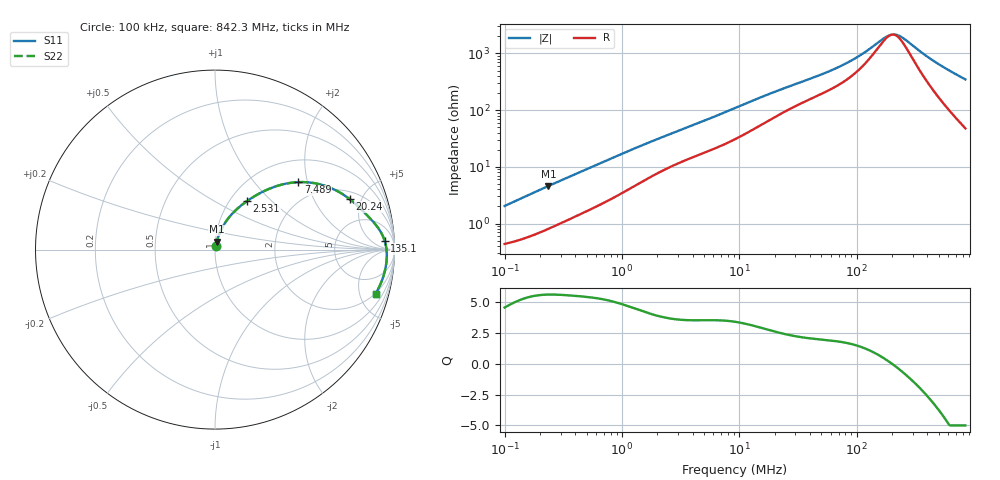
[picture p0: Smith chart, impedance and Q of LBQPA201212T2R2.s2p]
! LBQPA201212T2R2  S-PARAMETER MODEL  ( General Type )
! Model Generated by TAIYO YUDEN Corporation (http://www.ty-top.com)
! Version 1.0
! TAIYO YUDEN Control No. 191025NI43SB-FBB
! Copyright(c) 2019 TAIYO YUDEN CO.,LTD. All Rights Reserved.
! Product Description (link to TY-COMPAS)
! https://ds.yuden.co.jp/TYCOMPAS/or/detail?pn=LBQPA201212T2R2M&u=M
! Products Name : Inductors
! Characteristics :
!  Inductance : 2.2 uH , SRF(min) : 70 MHz , DC Resistance(max) : 0.429 Ohm
!  Rated Current : Saturation :530 mA , Temp Rise : 485 mA (20 degC)
!  Case Size : 2.0 x 1.25 / 0.079 x 0.049 [mm/inch] , Thickness : 1.25 / 0.049 [mm/inch]
!  (Conditions: Temperature = 25 degC , DC Bias Current/Voltage = 0A / 0V)
! External Node Assignments :
!  1  o---GGG---o  2
! GND o---------o GND
! Frequency Range : 0.1MHz  -  842.342835MHz  [ 402 STEP ]
# MHz S RI R 50
! Freq[MHz].  S11 Real  S11 Imag  S21 Real  S21 Imag  S12 Real  S12 Imag  S22 Real  S22 Imag
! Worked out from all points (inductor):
!   401 points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, 100 kHz to 842.3 MHz, reference 50 ohm
!   read as one part in series: L = 3.15 uH near 104.6 kHz
!   highest Q = 5.61 at 236 kHz (marker M1), where L = 3.05 uH
!   self-resonance near 199.7 MHz
!   S11 on the Smith chart (normalised r, x): 100 kHz: 1.01, +0.04; 2.531 MHz: 1.20, +0.72; 7.489 MHz: 1.50, +1.76; 20.24 MHz: 2.53, +3.97; 135.1 MHz: 19, +18; 842.3 MHz: 1.95, -6.91
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0.1  0.00474 0.0197  0.9953 -0.0197  0.9953 -0.0197  0.00474 0.0197
0.236005  0.00997 0.0444  0.99 -0.0444  0.99 -0.0444  0.00997 0.0444
0.454485  0.0212 0.0791  0.9788 -0.0791  0.9788 -0.0791  0.0212 0.0791
1.048642  0.0613 0.157  0.9387 -0.157  0.9387 -0.157  0.0613 0.157
2.065565  0.1428 0.2435  0.8572 -0.2435  0.8572 -0.2435  0.1428 0.2435
2.531409  0.1778 0.27  0.8222 -0.27  0.8222 -0.27  0.1778 0.27
4.354032  0.298 0.337  0.702 -0.337  0.702 -0.337  0.298 0.337
7.48895  0.4642 0.3759  0.5358 -0.3759  0.5358 -0.3759  0.4642 0.3759
9.177924  0.5333 0.3732  0.4667 -0.3732  0.4667 -0.3732  0.5333 0.3732
13.78451  0.6601 0.3369  0.3399 -0.3369  0.3399 -0.3369  0.6601 0.3369
20.24066  0.7498 0.2816  0.2502 -0.2816  0.2502 -0.2816  0.7498 0.2816
41.71227  0.8532 0.1854  0.1468 -0.1854  0.1468 -0.1854  0.8532 0.1854
80.32704  0.9156 0.111  0.0844 -0.111  0.0844 -0.111  0.9156 0.111
105.348  0.9336 0.0788  0.0664 -0.0788  0.0664 -0.0788  0.9336 0.0788
135.0757  0.9455 0.0486  0.0545 -0.0486  0.0545 -0.0486  0.9455 0.0486
169.3225  0.9525 0.0208  0.0475 -0.0208  0.0475 -0.0208  0.9525 0.0208
189.5759  0.9548 0.00662  0.0452 -0.00662  0.0452 -0.00662  0.9548 0.00662
212.252  0.9563 -0.00776  0.0437 0.00776  0.0437 0.00776  0.9563 -0.00776
237.6405  0.9571 -0.0224  0.0429 0.0224  0.0429 0.0224  0.9571 -0.0224
457.6341  0.9462 -0.12  0.0538 0.12  0.0538 0.12  0.9462 -0.12
642.2797  0.9253 -0.1844  0.0747 0.1844  0.0747 0.1844  0.9253 -0.1844
842.3428  0.8953 -0.2448  0.1047 0.2448  0.1047 0.2448  0.8953 -0.2448
